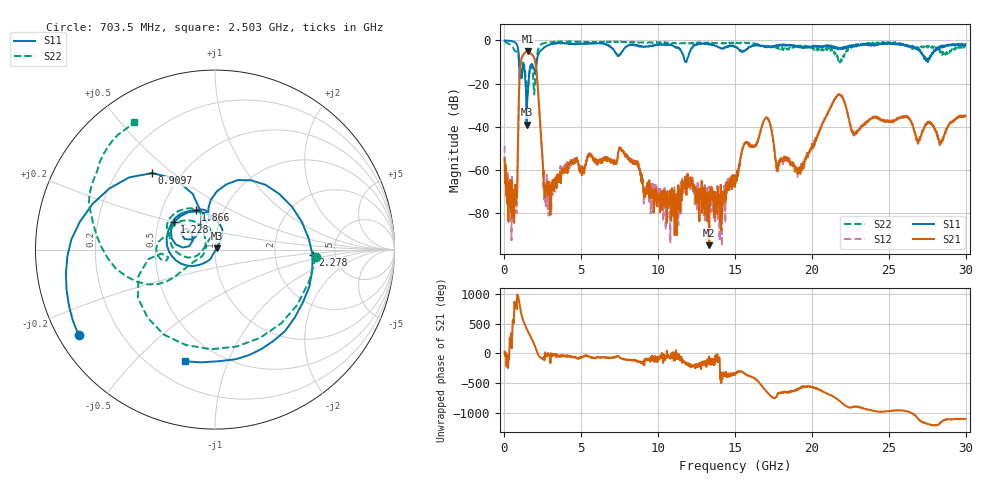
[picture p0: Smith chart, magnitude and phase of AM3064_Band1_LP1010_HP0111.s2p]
# Hz S DB R 50.0
!freq dBS11 angS11 dBS21 angS21 dBS12 angS12 dBS22 angS22
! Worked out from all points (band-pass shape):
!   1600 points, 10 MHz to 29.98 GHz, reference 50 ohm
!   highest |S21| = -5.12 dB at 1.51 GHz (marker M1); lowest = -95.0 dB at 13.32 GHz (marker M2)
!   |S21| within 3 dB of the highest: 1.123 GHz to 1.932 GHz (809.3 MHz wide, 53 % of centre)
!   lowest |S11| = -39.0 dB at 1.435 GHz (marker M3), VSWR 1.02, Z = 50.9 + j0.733 ohm
!   |S11| at or under -10 dB: 949.5 MHz to 2.106 GHz (1.157 GHz wide, 75.7 % of centre); 11.80404 GHz to 11.83984 GHz (35.8 MHz wide, 0.303 % of centre); 27.53984 GHz to 27.54521 GHz (5.372 MHz wide, 0.0195 % of centre)
!   |S22| runs from -25.0 to -0.3 dB; largest |S21 - S12| = 0.0065
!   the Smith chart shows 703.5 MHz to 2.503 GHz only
!   S11 on the Smith chart (normalised r, x): 703.5 MHz: 0.06, -0.29; 909.7 MHz: 0.35, +0.43; 1.228 GHz: 0.60, +0.20; 1.866 GHz: 0.74, +0.34; 2.278 GHz: 3.36, -0.27; 2.503 GHz: 0.33, -0.71
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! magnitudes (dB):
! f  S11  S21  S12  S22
! 10 MHz  0.0  -54.7  -48.8  -0.3
! 703.5 MHz  -0.9  -66.8  -67.1  -5.0
! 909.7 MHz  -5.2  -35.9  -35.8  -6.9
! 1.228 GHz  -11.2  -6.7  -6.6  -10.4
! 1.435 GHz  -39.0  -5.2  -5.1  -22.7
! 1.51 GHz  -25.3  -5.1  -5.1  -24.2
! 1.866 GHz  -12.3  -7.2  -7.1  -16.8
! 2.278 GHz  -5.3  -33.5  -33.4  -2.5
! 2.503 GHz  -3.8  -58.4  -56.8  -1.5
! 2.934 GHz  -1.9  -69.2  -71.6  -0.9
! 5.015 GHz  -1.5  -58.9  -61.7  -0.7
! 7.582 GHz  -6.2  -50.5  -50.5  -0.7
! 10 GHz  -2.0  -70.9  -69.0  -1.0
! 13.32 GHz  -1.6  -95.0  -67.7  -1.2
! 15 GHz  -3.0  -62.8  -63.7  -1.5
! 17.01 GHz  -3.2  -35.9  -35.8  -3.1
! 17.78 GHz  -2.3  -59.3  -61.8  -3.7
! 19.99 GHz  -3.1  -49.1  -48.8  -3.2
! 21.72 GHz  -3.7  -25.1  -25.1  -9.4
! 22.71 GHz  -2.2  -43.7  -43.7  -2.5
! 25 GHz  -1.1  -37.5  -37.0  -1.0
! 29.98 GHz  -1.8  -35.0  -35.2  -3.1
